(* Logix 5000 AddOnInstructionDefinition export Banner_LTF_Param_v4; software revision 33.00 *)

TYPE Banner_IOL_Port_v4 :   // UDT that has all of the data items necessary to communicate with a specific Port on a IO-Link Master
STRUCT
   Port_Controlled : INT;   // Each bit represents a port on an IO-Link Master. Set to 1 to tell AOI to control that port.
   Port_Activate : INT;   // Each bit represents a port on an IO-Link Master. When ON that port will process any commands in queue.
   Port_Read : INT;   // Each bit represents a port on an IO-Link Master. Used to determine when device AOI has requested a Read command.
   Port_Write : INT;   // Each bit represents a port on an IO-Link Master. Used to determine when device AOI has requested a Write command.
   Port_RW_Complete : INT;   // Each bit represents a port on an IO-Link Master. Tells device AOI that Read or Write request has been completed.
   Port_Device_Read : INT;
   Data_Transfer : SINT[190];   // Array to transfer data from IO-Master to device AOIs.
END_STRUCT
END_TYPE

TYPE Banner_LTF_RD_v4 :   // UDT with all of the Read only parameters for LTF.
STRUCT
   Master_Cycle_Time : INT;
   Min_Cycle_Time : INT;
   M_Sequence_Capability : INT;
   IO_Link_Version_ID : INT;
   Process_Data_Input_Length : INT;
   Process_Data_Output_Length : INT;
   Combined_Vendor_ID : DINT;   // IO-Link Vendor ID
   Vendor_ID1 : INT;
   Vendor_ID2 : INT;
   Combined_Device_ID : DINT;   // IO-Link Device ID
   Device_ID1 : INT;
   Device_ID2 : INT;
   Device_ID3 : INT;
   Serial_Number : STRING;
   Teach_State : SINT;   // 0 =IDLE, 1 = SP1 Success, 4 = Wait for Command, 5 = Busy, 7 = Error
   SP1_TP1 : SINT;   // 0 = not taught or unsuccessful, 1 = successfully taught
   SP2_TP2 : SINT;   // 0 = not taught or unsuccessful, 1 = successfully taught
   Measurement_Value : DINT;   // Measurement value in .1 mm.
   Excess_Gain_Percent : DINT;   // Excess gain expressed as a percentage of minimum signal
   Stability : INT;   // 0 = No target exists, 1 = Marginal or multiple peaks, 2 = Stable
   Display_String : STRING;   // String currently being displayed on the LED display of the sensor
END_STRUCT
END_TYPE

TYPE Banner_LTF_v4 :   // UDT with all of the parameters for LTF.
STRUCT
   Initial_Global_Read : BOOL;   // Determines if all of the IO-Link data has been read into the PLC yet
   Command : INT;   // Value placed in here will activate a read or write to a specifc IO-Link Index
   Read_Data : Banner_LTF_RD_v4;   // Read Only Data
   Write_Data : Banner_LTF_WD_v4;   // Write Data
   Archive : Banner_LTF_WD_v4;   // Archive write data
   Reset : BOOL;   // Resets AOI. This will force a complete parameter read of the sensor.
END_STRUCT
END_TYPE

TYPE Banner_LTF_WD_v4 :   // UDT that stores the Write Data for a LTF.
STRUCT
   System_Command : INT;   // See IODD file for list of commands that can be activated via the System Command interface
   Parameter_Access_Lock : SINT;   // Write access to all parameters is prohibited while value is 1. Only this parameter can be adjusted when value is 1.
   Data_Storage_Lock : SINT;   // Automatic data storage is disabled when this value is equal to 1. Read access is not affected.
   Local_Parameterization_Lock : SINT;   // Parameterization via local control elements on device is disabled.
   Local_User_Interface_Lock : SINT;   // Operation of local user interface is disabled.
   Teach_Channel : INT;   // 0 = Default, 1 = BDC1, 2 = BDC2
   BDC1_Setpoint_SP1 : DINT;   // SP1 switch point in Switch or Window mode. Range 500 to 120000 (.1 mm increments)
   BDC1_Setpoint_SP2 : DINT;   // SP2 switch point in Window mode only. Range 500 to 120000 (.1 mm increments)
   BDC1_Swithpoint_Logic : INT;   // Discrete output only. 0 = Light Operate, 1 = Dark Operate
   BDC1_BDC_Mode : INT;   // 1 = Switch Mode/Single Point Mode, 2 = Window Mode, 132 = Health(LO)/Alarm Mode(DO)
   BDC1_Hysteresis : DINT;   // 0 = Automatically set by sensor, 2-12000 = Manual (2 to 12000 mm)
   BDC2_Setpoint_SP1 : DINT;   // SP1 switch point in Switch or Window mode. Range 500 to 120000 (.1 mm increments)
   BDC2_Setpoint_SP2 : DINT;   // SP2 switch point in Window mode only. Range 500 to 120000 (.1 mm increments)
   BDC2_Switchpoint_Logic : INT;   // Discrete output only. 0 = Light Operate, 1 = Dark Operate
   BDC2_BDC_Mode : INT;   // 1 = Switch Mode/Single Point Mode, 2 = Window Mode, 132 = Health(LO)/Alarm Mode(DO), 133 Pulse Frequency Modulation
   BDC2_Hysteresis : DINT;   // 0 = Automatically set by sensor, 2-12000 = Manual (2 to 12000 mm)
   Response_Speed : INT;   // 0 = Fast, 1 = Standard, 2 = Medium, 3 = Slow
   Zero_Reference_Location : INT;   // 0 = Near, 1 = Far
   Shift_Zero_Reference_After_Teach : INT;   // 0 = Off, 1 = AutoSet, 2 = SetZero
   Sensor_Lockout : SINT;   // 0 = No Lock Out, 1 = Sensor Locked
   Output_Polarity : SINT;   // 0 = PNP, 1 = NPN
   IOL_Filter_Time : DINT;   // Time to average IOL process data measurement between updates. 0 to 65535 ms.
   Display_Read : SINT;   // 0 = Nomral, 1 = Inverted
   Display_Units : SINT;   // 0 = mm, 1 = inches
   Display_Sleep : SINT;   // 0 = 1 min, 1 = 5 min, 2 = 15 min, 3 = 60 min, 4 = Disabled
   Remote_Input_Type : SINT;   // 0 = Teach, 1 = Laser Enable, 2 = Sync Master, 3 = Sync Slave, 4 = Disabled
   BDC1_Delay_Mode : INT;   // 0 = Delay timer disabled, 1 = On & Off Delay, 2 = Off One-Shot timer, 3 = On One-Shot timer
   BDC1_Delay_On_OneShot_Delay : DINT;   // 0 to 9999 ms. 0 ms disables On delay or On/Off oneshot delay.
   BDC1_Delay_Off_OneShot_Delay : DINT;   // 0 to 9999 ms. 0 ms disables Off delay or On/Off oneshot delay.
   BDC1_Switch_Point_Reference : INT;   // 0 = Object, 1 = Background, 2 = Custom
   BDC1_User_Teach_Offset : DINT;   // The user selected teach offset. In Custom mode this value can be either + or -. In Object or Background mode this must be set to 0. Range -119500 to 119500 (-11950 to 11950 mm)
   BDC1_Midpoint_Window_Size : DINT;   // In Midpoint teach mode this will set the size of the window for midpoint teach. Default is 20 mm. Range 0 to 119500 (0 - 11950 mm).
   BDC1_Midpoint_Teach_Offset_Size : DINT;   // The offset value that is applied to a Midpoint teach. Range: -119500 to 119500 (-11950 to 11950 mm)
   BDC2_Delay_Mode : INT;   // 0 = Delay timer disabled, 1 = On & Off Delay, 2 = Off One-Shot timer, 3 = On One-Shot timer
   BDC2_Delay_On_OneShot_Delay : DINT;   // 0 to 9999. 0 ms disables On delay or On/Off oneshot delay.
   BDC2_Delay_Off_OneShot_Delay : DINT;   // 0 to 9999. 0 ms disables Off delay or On/Off oneshot delay.
   BDC2_Switch_Point_Reference : INT;   // 0 = Object, 1 = Background, 2 = Custom
   BDC2_User_Teach_Offset : DINT;   // The user selected teach offset. In Custom mode this value can be either + or -. In Object or Background mode this must be set to 0. Range: -119500 to 119500 (-11950 to 11950 mm).
   BDC2_Midpoint_Window_Size : DINT;   // In Midpoint teach mode this will set the size of the window for midpoint teach. Default is 20 mm. Range 0 to 119500 (0 - 11950 mm).
   BDC2_Midpoint_Teach_Offset_Size : DINT;   // The offset value that is applied to a Midpoint teach. Range: -119500 to 119500 (-11950 to 11950 mm).
   Near_Frequency : DINT;   // Frequency corresponding to a target at the near limit of the sensing range. Range 100 to 10000 Hz.
   Far_Frequency : DINT;   // Frequency corresponding to a target at the far limit of the sensing range. Range 100 to 10000 Hz.
END_STRUCT
END_TYPE

ADD_ON_INSTRUCTION Banner_LTF_Param_v4   (* revision 4.1, vendor Banner Engineering *)
// AOI to read and write parameter data to an IO-Link LTF.
VAR_IN_OUT
   LTF : Banner_LTF_v4; {required}
   Port_Data : Banner_IOL_Port_v4; {required}
END_VAR
VAR_INPUT
   Port : DINT; {required}
END_VAR
VAR
   Local_Control : DINT; {access None}
   Global_Read_Command_Value : INT; {access None}
   Global_Write_Command_Value : INT; {access None}
   Command_Being_Processed : BOOL; {access None}
   Update_Archive : BOOL; {access None}
   Index_Write_Control : DINT; {access None}
   Index_Write_Inprocess : INT; {access None}
   Inprocess_Index : DINT; {access None}
END_VAR

ROUTINE Logic   (* ladder *)
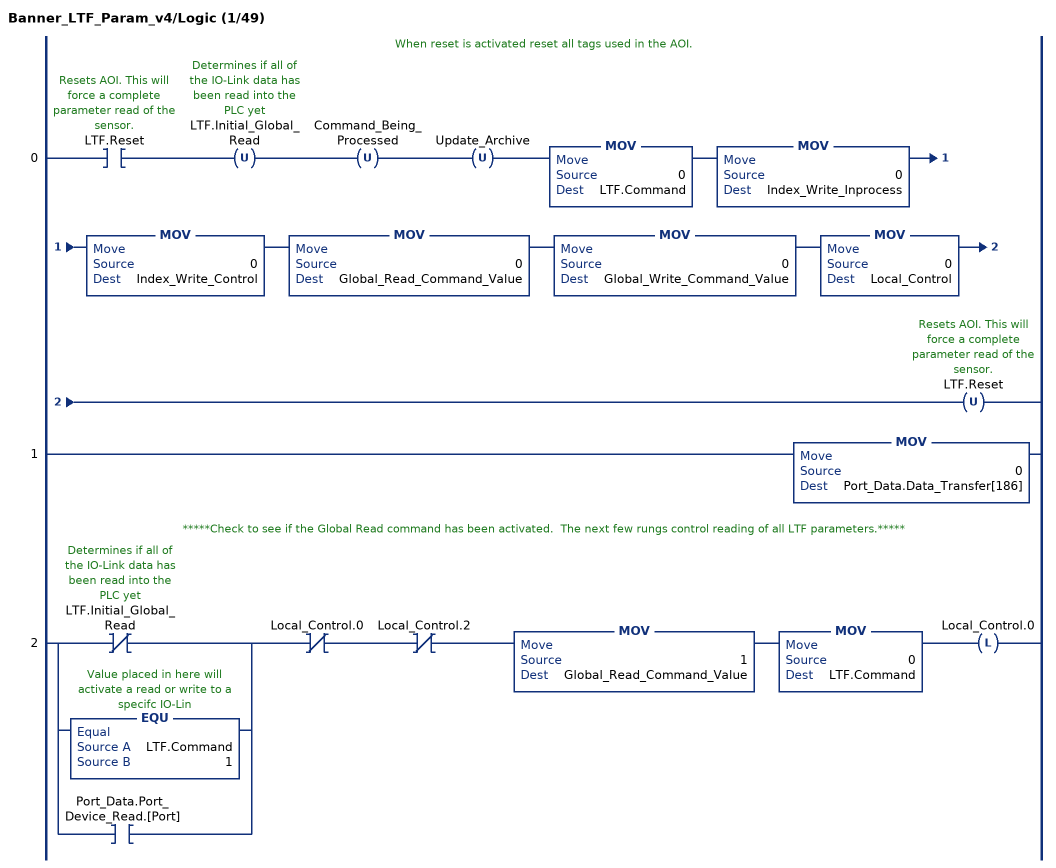
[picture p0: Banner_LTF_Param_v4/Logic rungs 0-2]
   // When reset is activated reset all tags used in the AOI.
   0: XIC(LTF.Reset)OTU(LTF.Initial_Global_Read)OTU(Command_Being_Processed)OTU(Update_Archive)MOV(0,LTF.Command)MOV(0,Index_Write_Inprocess)MOV(0,Index_Write_Control)MOV(0,Global_Read_Command_Value)MOV(0,Global_Write_Command_Value)MOV(0,Local_Control)OTU(LTF.Reset);
   1: MOV(0,Port_Data.Data_Transfer[186]);
   // *****Check to see if the Global Read command has been activated.  The next few rungs control reading of all LTF parameters.*****
   2: [XIO(LTF.Initial_Global_Read) ,EQU(LTF.Command,1) ,XIC(Port_Data.Port_Device_Read.[Port]) ]XIO(Local_Control.0)XIO(Local_Control.2)MOV(1,Global_Read_Command_Value)MOV(0,LTF.Command)OTL(Local_Control.0);
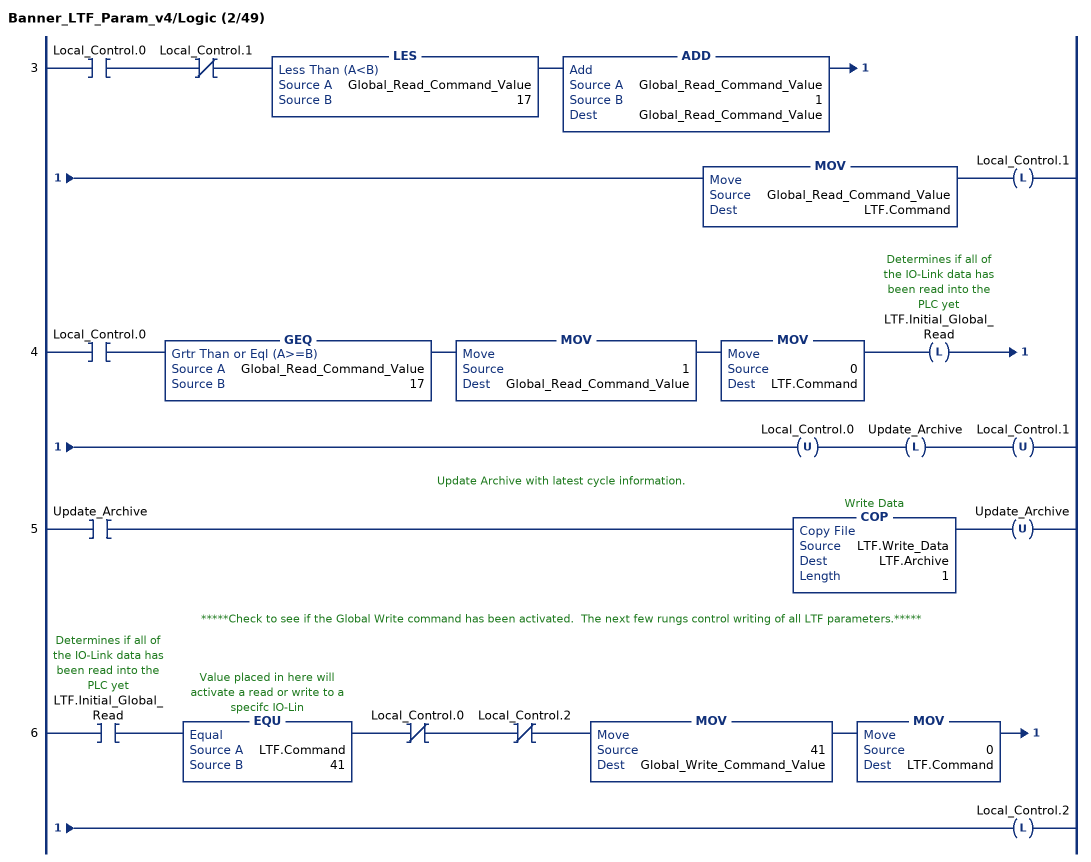
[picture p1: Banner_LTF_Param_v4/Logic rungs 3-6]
   3: XIC(Local_Control.0)XIO(Local_Control.1)LES(Global_Read_Command_Value,17)ADD(Global_Read_Command_Value,1,Global_Read_Command_Value)MOV(Global_Read_Command_Value,LTF.Command)OTL(Local_Control.1);
   4: XIC(Local_Control.0)GEQ(Global_Read_Command_Value,17)MOV(1,Global_Read_Command_Value)MOV(0,LTF.Command)OTL(LTF.Initial_Global_Read)OTU(Local_Control.0)OTL(Update_Archive)OTU(Local_Control.1);
   // Update Archive with latest cycle information.
   5: XIC(Update_Archive)COP(LTF.Write_Data,LTF.Archive,1)OTU(Update_Archive);
   // *****Check to see if the Global Write command has been activated.  The next few rungs control writing of all LTF parameters.*****
   6: XIC(LTF.Initial_Global_Read)EQU(LTF.Command,41)XIO(Local_Control.0)XIO(Local_Control.2)MOV(41,Global_Write_Command_Value)MOV(0,LTF.Command)OTL(Local_Control.2);
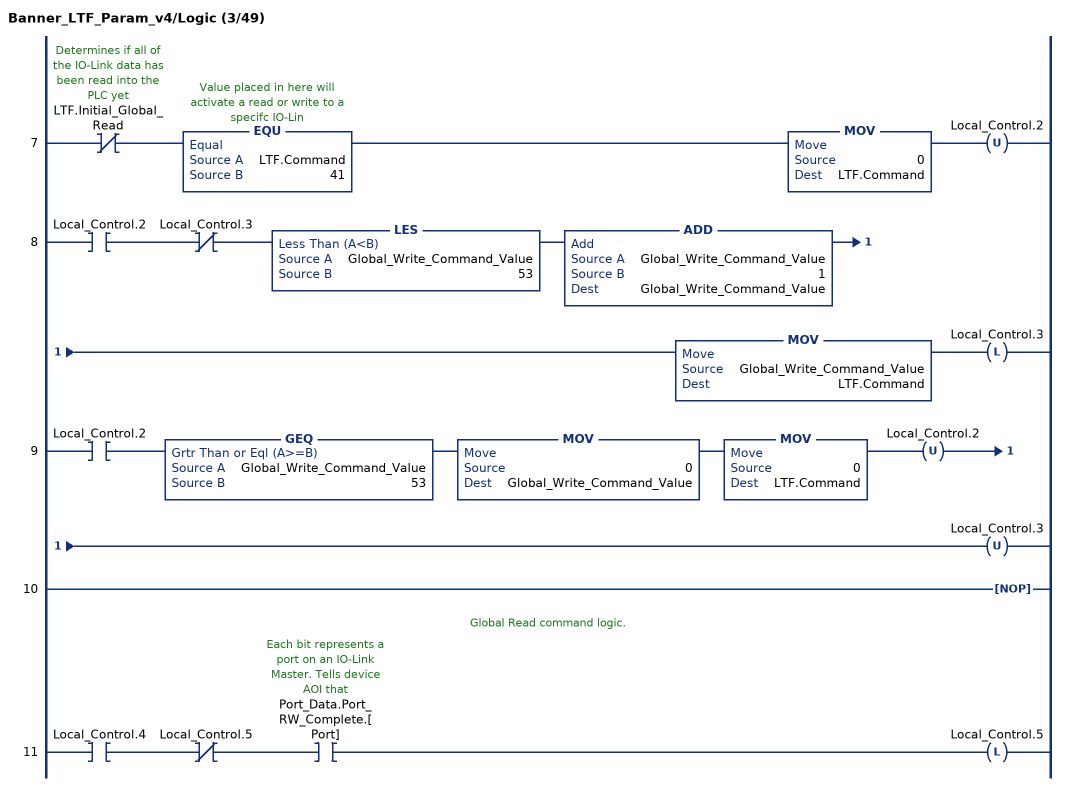
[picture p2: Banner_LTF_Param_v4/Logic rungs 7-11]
   7: XIO(LTF.Initial_Global_Read)EQU(LTF.Command,41)MOV(0,LTF.Command)OTU(Local_Control.2);
   8: XIC(Local_Control.2)XIO(Local_Control.3)LES(Global_Write_Command_Value,53)ADD(Global_Write_Command_Value,1,Global_Write_Command_Value)MOV(Global_Write_Command_Value,LTF.Command)OTL(Local_Control.3);
   9: XIC(Local_Control.2)GEQ(Global_Write_Command_Value,53)MOV(0,Global_Write_Command_Value)MOV(0,LTF.Command)OTU(Local_Control.2)OTU(Local_Control.3);
   10: NOP();
   // Global Read command logic.
   11: XIC(Local_Control.4)XIO(Local_Control.5)XIC(Port_Data.Port_RW_Complete.[Port])OTL(Local_Control.5);
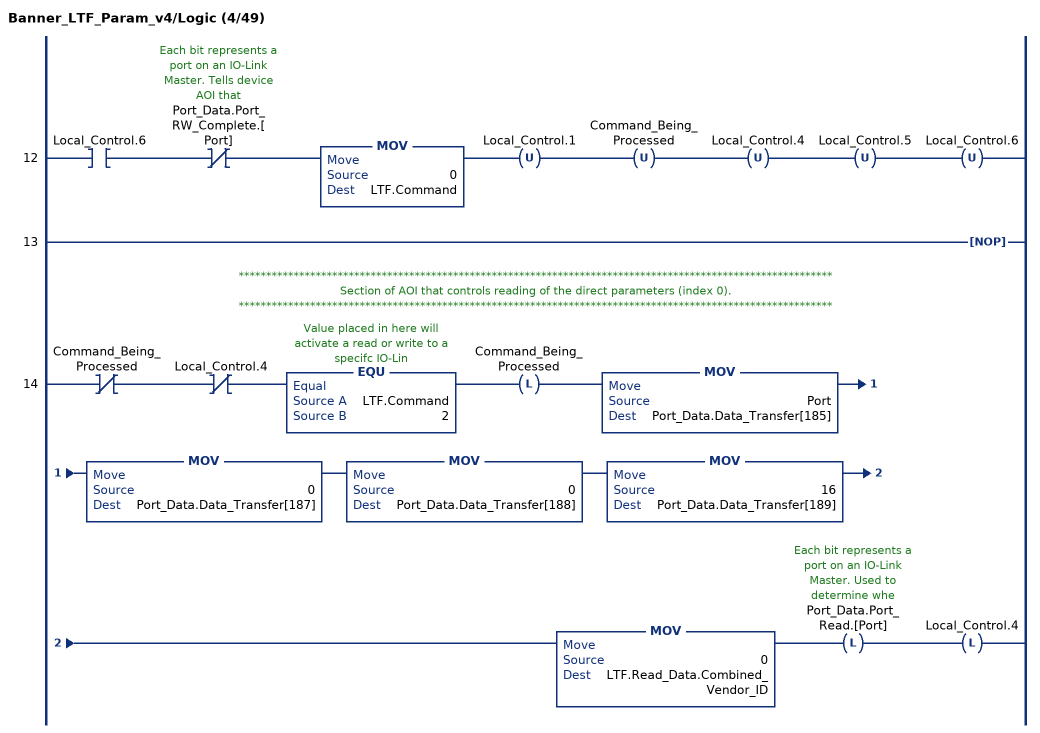
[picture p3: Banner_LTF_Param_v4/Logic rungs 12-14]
   12: XIC(Local_Control.6)XIO(Port_Data.Port_RW_Complete.[Port])MOV(0,LTF.Command)OTU(Local_Control.1)OTU(Command_Being_Processed)OTU(Local_Control.4)OTU(Local_Control.5)OTU(Local_Control.6);
   13: NOP();
   // ************************************************************************************************************
   // Section of AOI that controls reading of the direct parameters (index 0).
   // ************************************************************************************************************
   14: XIO(Command_Being_Processed)XIO(Local_Control.4)EQU(LTF.Command,2)OTL(Command_Being_Processed)MOV(Port,Port_Data.Data_Transfer[185])MOV(0,Port_Data.Data_Transfer[187])MOV(0,Port_Data.Data_Transfer[188])MOV(16,Port_Data.Data_Transfer[189])MOV(0,LTF.Read_Data.Combined_Vendor_ID)OTL(Port_Data.Port_Read.[Port])OTL(Local_Control.4);
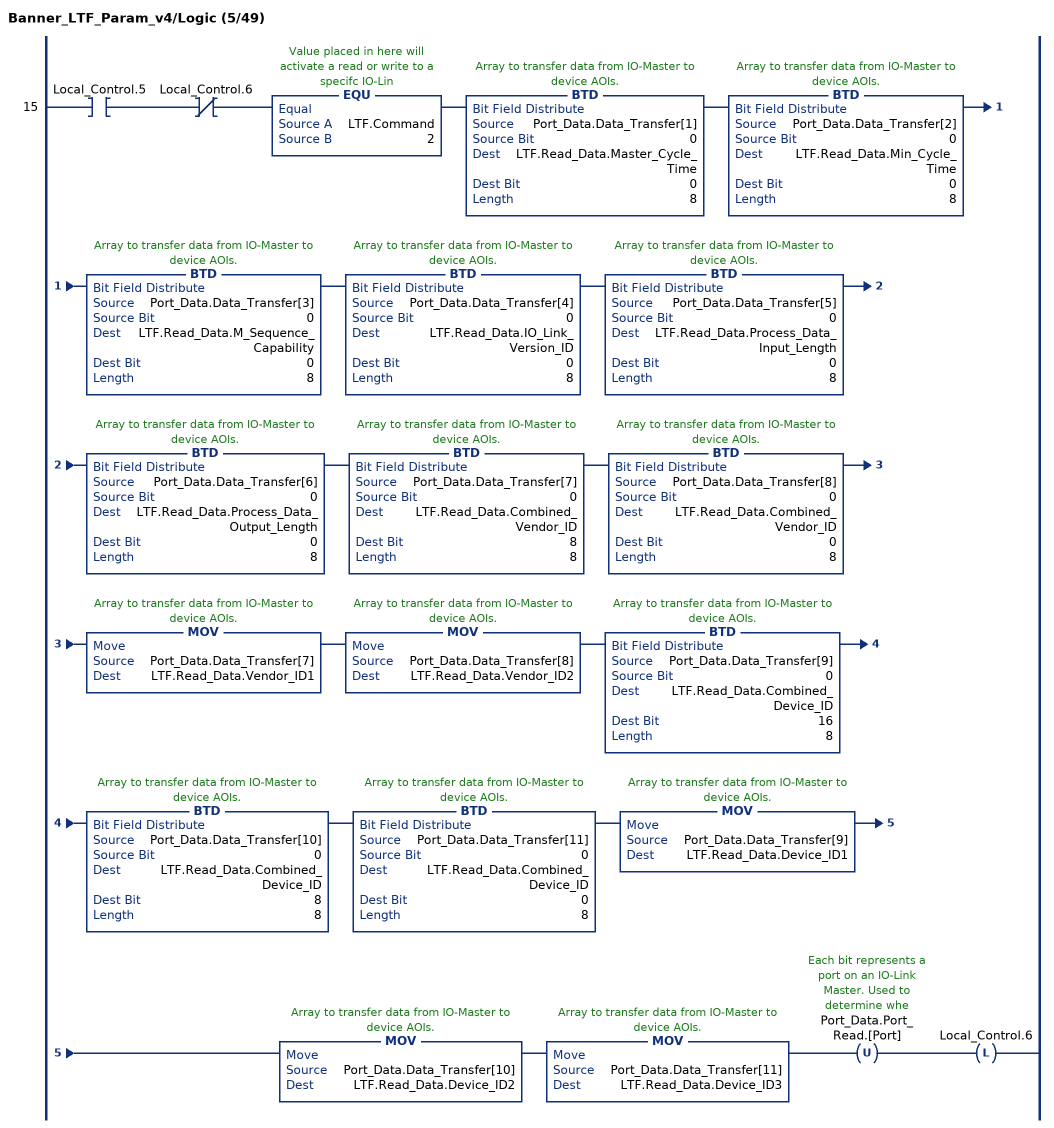
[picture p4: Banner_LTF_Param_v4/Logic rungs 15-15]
   15: XIC(Local_Control.5)XIO(Local_Control.6)EQU(LTF.Command,2)BTD(Port_Data.Data_Transfer[1],0,LTF.Read_Data.Master_Cycle_Time,0,8)BTD(Port_Data.Data_Transfer[2],0,LTF.Read_Data.Min_Cycle_Time,0,8)BTD(Port_Data.Data_Transfer[3],0,LTF.Read_Data.M_Sequence_Capability,0,8)BTD(Port_Data.Data_Transfer[4],0,LTF.Read_Data.IO_Link_Version_ID,0,8)BTD(Port_Data.Data_Transfer[5],0,LTF.Read_Data.Process_Data_Input_Length,0,8)BTD(Port_Data.Data_Transfer[6],0,LTF.Read_Data.Process_Data_Output_Length,0,8)BTD(Port_Data.Data_Transfer[7],0,LTF.Read_Data.Combined_Vendor_ID,8,8)BTD(Port_Data.Data_Transfer[8],0,LTF.Read_Data.Combined_Vendor_ID,0,8)MOV(Port_Data.Data_Transfer[7],LTF.Read_Data.Vendor_ID1)MOV(Port_Data.Data_Transfer[8],LTF.Read_Data.Vendor_ID2)BTD(Port_Data.Data_Transfer[9],0,LTF.Read_Data.Combined_Device_ID,16,8)BTD(Port_Data.Data_Transfer[10],0,LTF.Read_Data.Combined_Device_ID,8,8)BTD(Port_Data.Data_Transfer[11],0,LTF.Read_Data.Combined_Device_ID,0,8)MOV(Port_Data.Data_Transfer[9],LTF.Read_Data.Device_ID1)MOV(Port_Data.Data_Transfer[10],LTF.Read_Data.Device_ID2)MOV(Port_Data.Data_Transfer[11],LTF.Read_Data.Device_ID3)OTU(Port_Data.Port_Read.[Port])OTL(Local_Control.6);
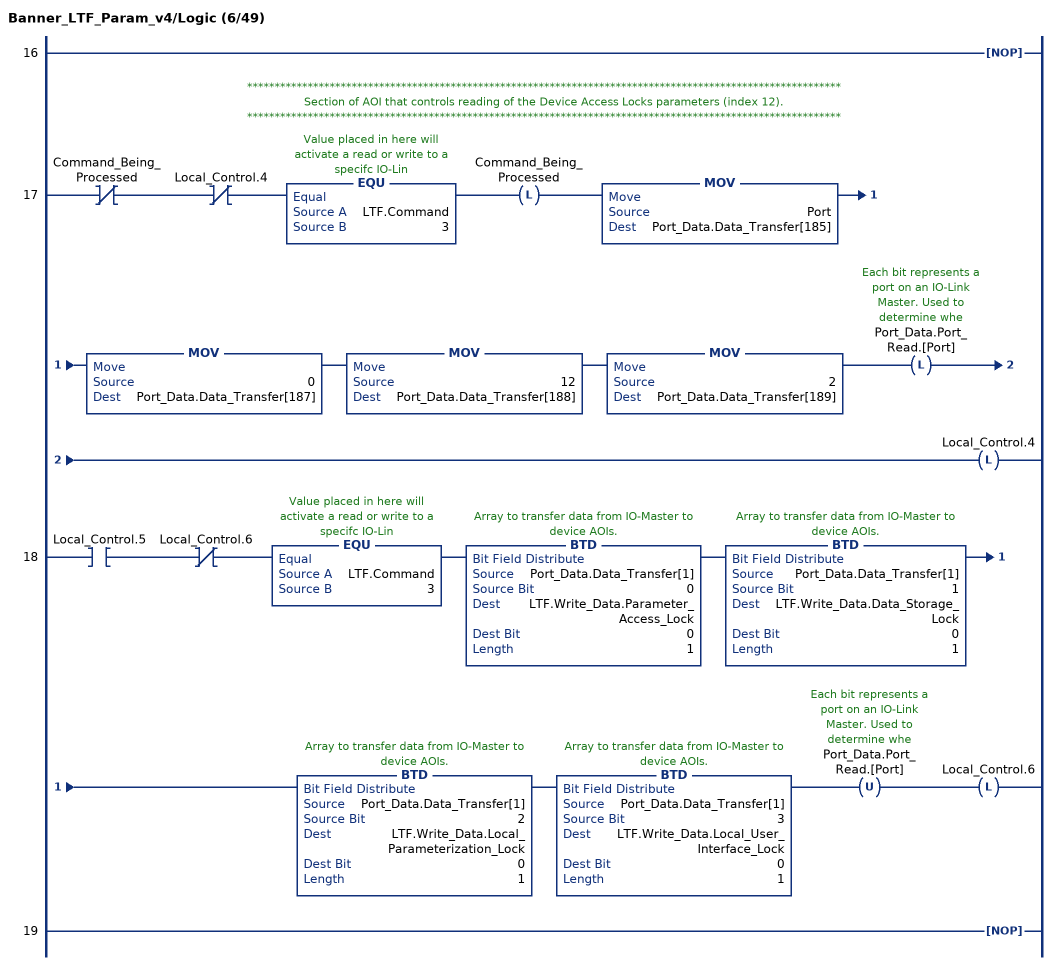
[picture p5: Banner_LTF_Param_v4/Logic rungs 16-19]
   16: NOP();
   // ************************************************************************************************************
   // Section of AOI that controls reading of the Device Access Locks parameters (index 12).
   // ************************************************************************************************************
   17: XIO(Command_Being_Processed)XIO(Local_Control.4)EQU(LTF.Command,3)OTL(Command_Being_Processed)MOV(Port,Port_Data.Data_Transfer[185])MOV(0,Port_Data.Data_Transfer[187])MOV(12,Port_Data.Data_Transfer[188])MOV(2,Port_Data.Data_Transfer[189])OTL(Port_Data.Port_Read.[Port])OTL(Local_Control.4);
   18: XIC(Local_Control.5)XIO(Local_Control.6)EQU(LTF.Command,3)BTD(Port_Data.Data_Transfer[1],0,LTF.Write_Data.Parameter_Access_Lock,0,1)BTD(Port_Data.Data_Transfer[1],1,LTF.Write_Data.Data_Storage_Lock,0,1)BTD(Port_Data.Data_Transfer[1],2,LTF.Write_Data.Local_Parameterization_Lock,0,1)BTD(Port_Data.Data_Transfer[1],3,LTF.Write_Data.Local_User_Interface_Lock,0,1)OTU(Port_Data.Port_Read.[Port])OTL(Local_Control.6);
   19: NOP();
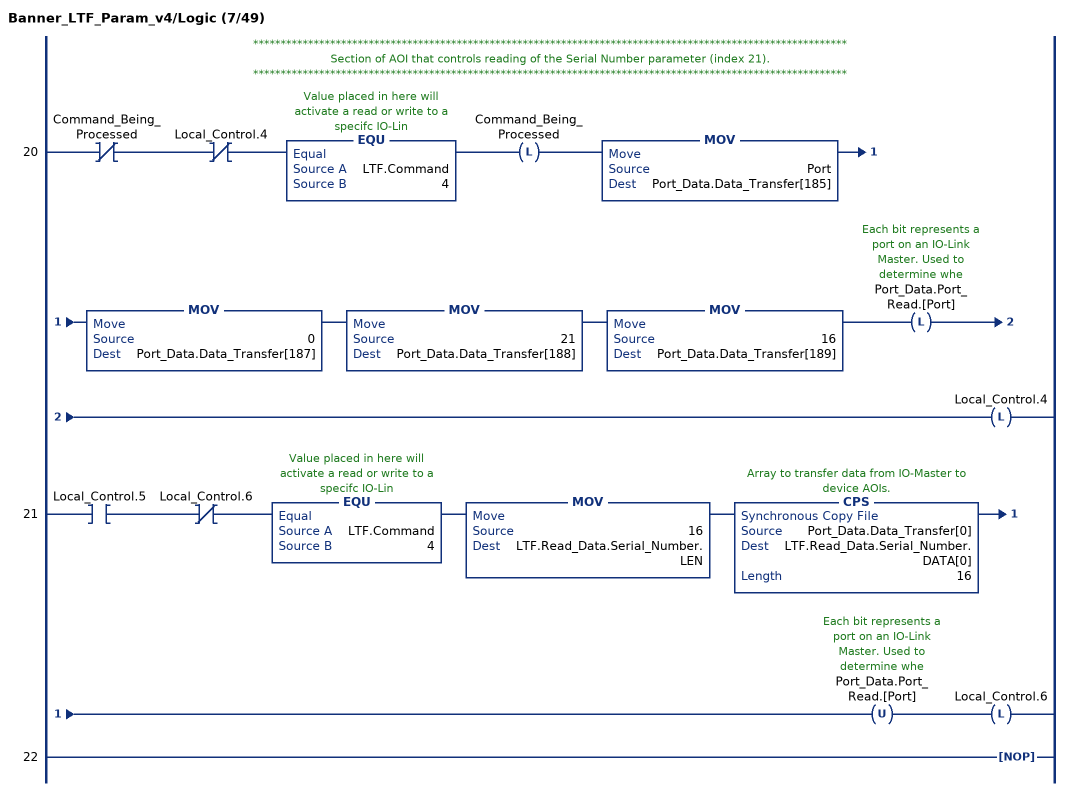
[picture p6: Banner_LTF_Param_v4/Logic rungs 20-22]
   // ************************************************************************************************************
   // Section of AOI that controls reading of the Serial Number parameter (index 21).
   // ************************************************************************************************************
   20: XIO(Command_Being_Processed)XIO(Local_Control.4)EQU(LTF.Command,4)OTL(Command_Being_Processed)MOV(Port,Port_Data.Data_Transfer[185])MOV(0,Port_Data.Data_Transfer[187])MOV(21,Port_Data.Data_Transfer[188])MOV(16,Port_Data.Data_Transfer[189])OTL(Port_Data.Port_Read.[Port])OTL(Local_Control.4);
   21: XIC(Local_Control.5)XIO(Local_Control.6)EQU(LTF.Command,4)MOV(16,LTF.Read_Data.Serial_Number.LEN)CPS(Port_Data.Data_Transfer[0],LTF.Read_Data.Serial_Number.DATA[0],16)OTU(Port_Data.Port_Read.[Port])OTL(Local_Control.6);
   22: NOP();
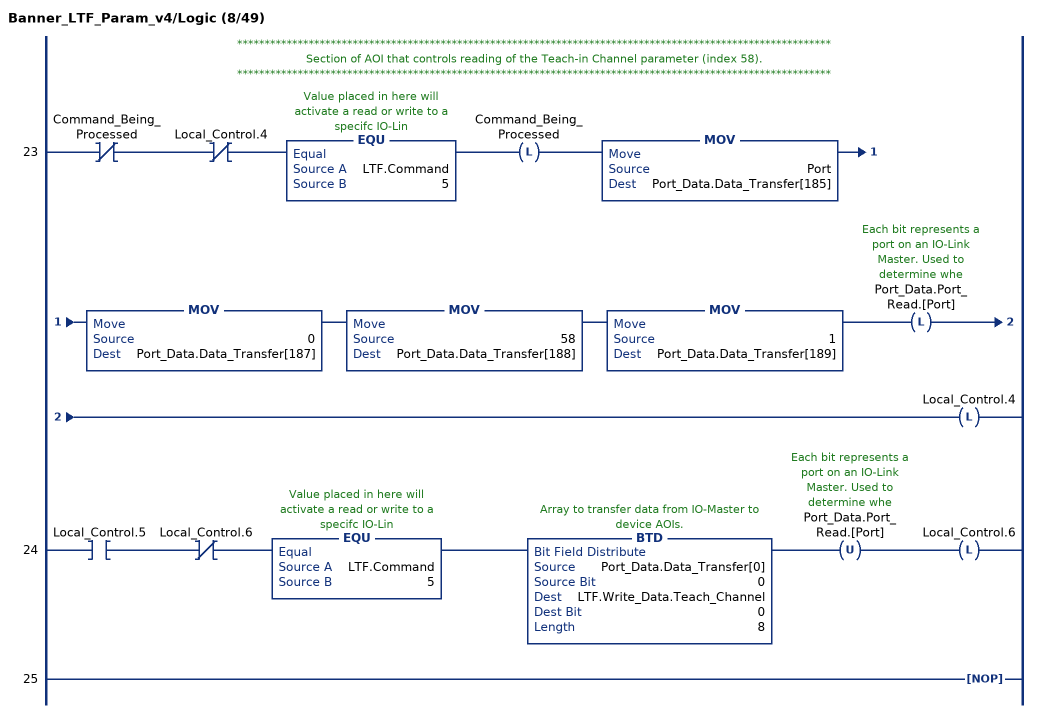
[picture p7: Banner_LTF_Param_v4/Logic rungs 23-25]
   // ************************************************************************************************************
   // Section of AOI that controls reading of the Teach-in Channel parameter (index 58).
   // ************************************************************************************************************
   23: XIO(Command_Being_Processed)XIO(Local_Control.4)EQU(LTF.Command,5)OTL(Command_Being_Processed)MOV(Port,Port_Data.Data_Transfer[185])MOV(0,Port_Data.Data_Transfer[187])MOV(58,Port_Data.Data_Transfer[188])MOV(1,Port_Data.Data_Transfer[189])OTL(Port_Data.Port_Read.[Port])OTL(Local_Control.4);
   24: XIC(Local_Control.5)XIO(Local_Control.6)EQU(LTF.Command,5)BTD(Port_Data.Data_Transfer[0],0,LTF.Write_Data.Teach_Channel,0,8)OTU(Port_Data.Port_Read.[Port])OTL(Local_Control.6);
   25: NOP();
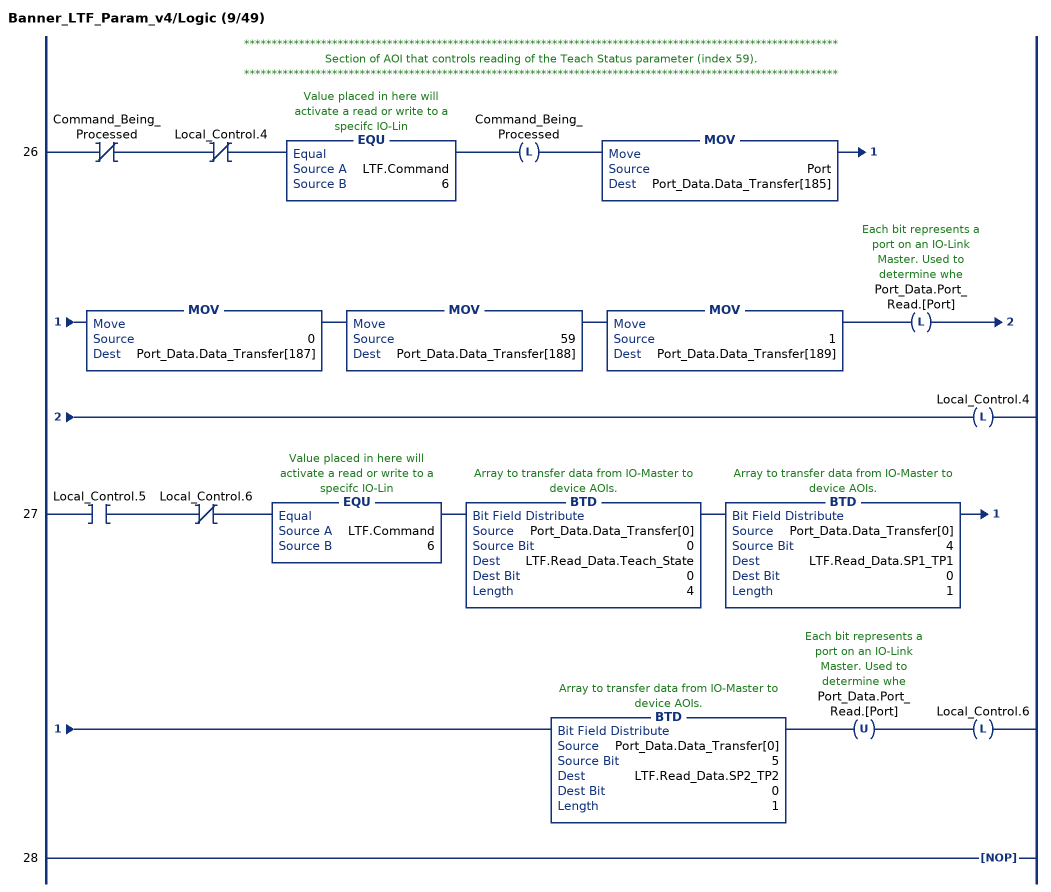
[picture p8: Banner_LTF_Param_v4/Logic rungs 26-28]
   // ************************************************************************************************************
   // Section of AOI that controls reading of the Teach Status parameter (index 59).
   // ************************************************************************************************************
   26: XIO(Command_Being_Processed)XIO(Local_Control.4)EQU(LTF.Command,6)OTL(Command_Being_Processed)MOV(Port,Port_Data.Data_Transfer[185])MOV(0,Port_Data.Data_Transfer[187])MOV(59,Port_Data.Data_Transfer[188])MOV(1,Port_Data.Data_Transfer[189])OTL(Port_Data.Port_Read.[Port])OTL(Local_Control.4);
   27: XIC(Local_Control.5)XIO(Local_Control.6)EQU(LTF.Command,6)BTD(Port_Data.Data_Transfer[0],0,LTF.Read_Data.Teach_State,0,4)BTD(Port_Data.Data_Transfer[0],4,LTF.Read_Data.SP1_TP1,0,1)BTD(Port_Data.Data_Transfer[0],5,LTF.Read_Data.SP2_TP2,0,1)OTU(Port_Data.Port_Read.[Port])OTL(Local_Control.6);
   28: NOP();
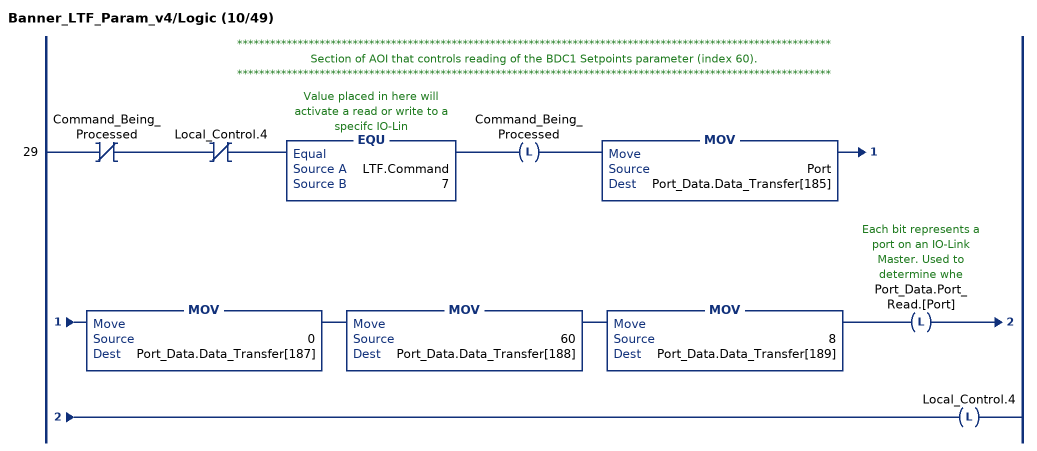
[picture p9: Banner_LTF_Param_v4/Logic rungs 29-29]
   // ************************************************************************************************************
   // Section of AOI that controls reading of the BDC1 Setpoints parameter (index 60).
   // ************************************************************************************************************
   29: XIO(Command_Being_Processed)XIO(Local_Control.4)EQU(LTF.Command,7)OTL(Command_Being_Processed)MOV(Port,Port_Data.Data_Transfer[185])MOV(0,Port_Data.Data_Transfer[187])MOV(60,Port_Data.Data_Transfer[188])MOV(8,Port_Data.Data_Transfer[189])OTL(Port_Data.Port_Read.[Port])OTL(Local_Control.4);
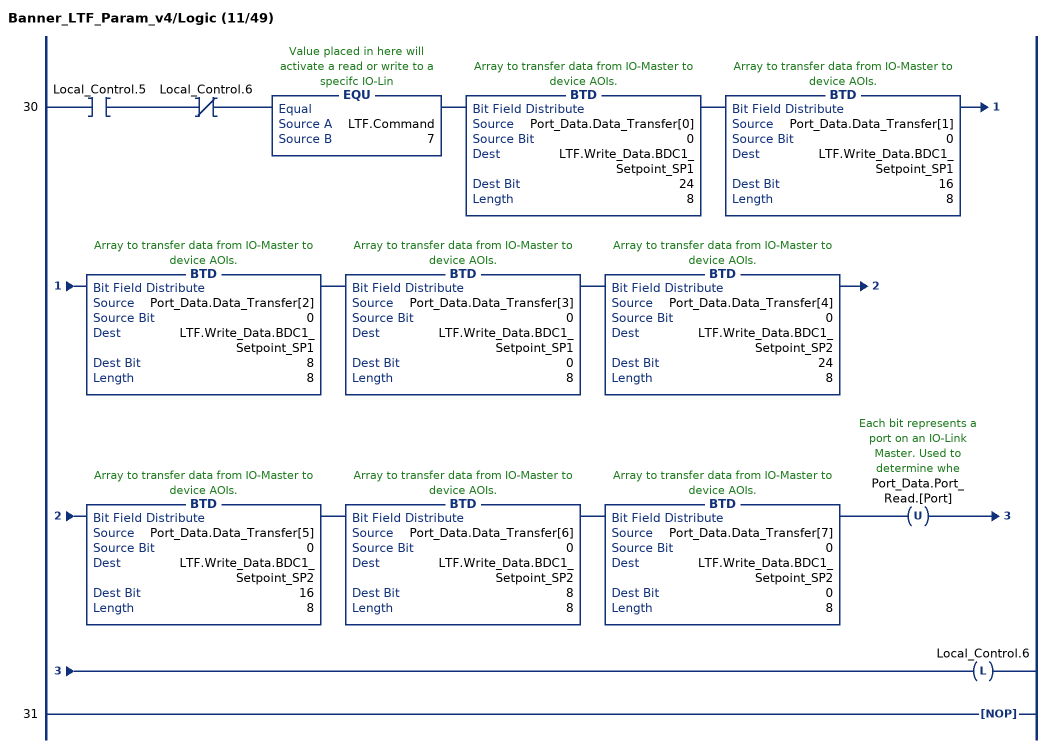
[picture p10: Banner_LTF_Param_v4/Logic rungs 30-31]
   30: XIC(Local_Control.5)XIO(Local_Control.6)EQU(LTF.Command,7)BTD(Port_Data.Data_Transfer[0],0,LTF.Write_Data.BDC1_Setpoint_SP1,24,8)BTD(Port_Data.Data_Transfer[1],0,LTF.Write_Data.BDC1_Setpoint_SP1,16,8)BTD(Port_Data.Data_Transfer[2],0,LTF.Write_Data.BDC1_Setpoint_SP1,8,8)BTD(Port_Data.Data_Transfer[3],0,LTF.Write_Data.BDC1_Setpoint_SP1,0,8)BTD(Port_Data.Data_Transfer[4],0,LTF.Write_Data.BDC1_Setpoint_SP2,24,8)BTD(Port_Data.Data_Transfer[5],0,LTF.Write_Data.BDC1_Setpoint_SP2,16,8)BTD(Port_Data.Data_Transfer[6],0,LTF.Write_Data.BDC1_Setpoint_SP2,8,8)BTD(Port_Data.Data_Transfer[7],0,LTF.Write_Data.BDC1_Setpoint_SP2,0,8)OTU(Port_Data.Port_Read.[Port])OTL(Local_Control.6);
   31: NOP();
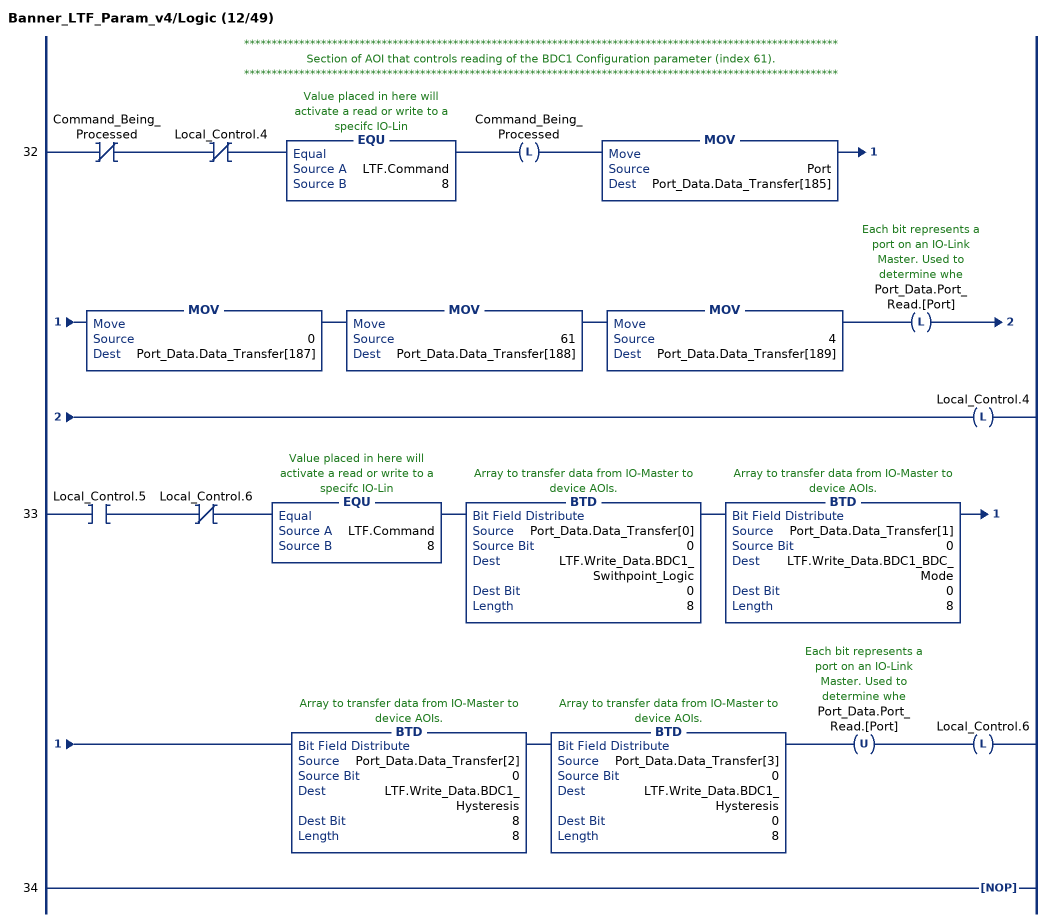
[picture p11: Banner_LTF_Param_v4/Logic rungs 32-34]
   // ************************************************************************************************************
   // Section of AOI that controls reading of the BDC1 Configuration parameter (index 61).
   // ************************************************************************************************************
   32: XIO(Command_Being_Processed)XIO(Local_Control.4)EQU(LTF.Command,8)OTL(Command_Being_Processed)MOV(Port,Port_Data.Data_Transfer[185])MOV(0,Port_Data.Data_Transfer[187])MOV(61,Port_Data.Data_Transfer[188])MOV(4,Port_Data.Data_Transfer[189])OTL(Port_Data.Port_Read.[Port])OTL(Local_Control.4);
   33: XIC(Local_Control.5)XIO(Local_Control.6)EQU(LTF.Command,8)BTD(Port_Data.Data_Transfer[0],0,LTF.Write_Data.BDC1_Swithpoint_Logic,0,8)BTD(Port_Data.Data_Transfer[1],0,LTF.Write_Data.BDC1_BDC_Mode,0,8)BTD(Port_Data.Data_Transfer[2],0,LTF.Write_Data.BDC1_Hysteresis,8,8)BTD(Port_Data.Data_Transfer[3],0,LTF.Write_Data.BDC1_Hysteresis,0,8)OTU(Port_Data.Port_Read.[Port])OTL(Local_Control.6);
   34: NOP();
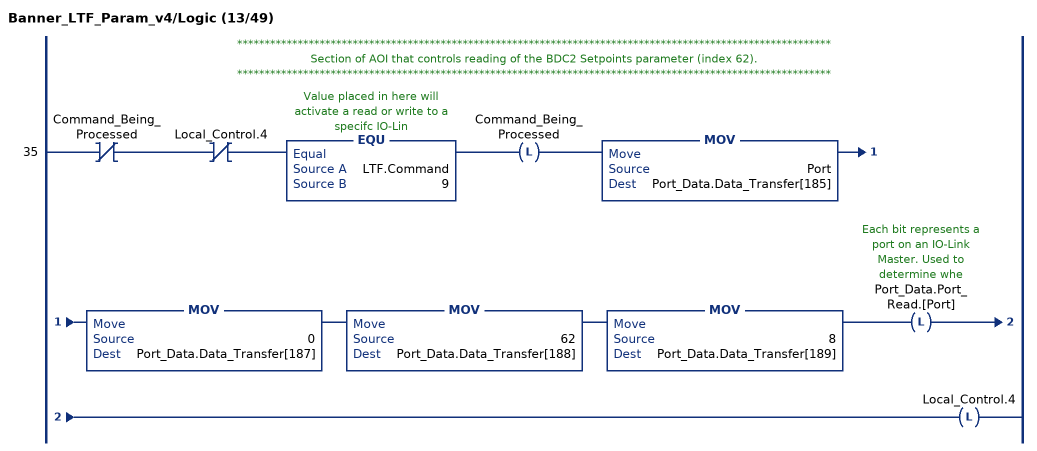
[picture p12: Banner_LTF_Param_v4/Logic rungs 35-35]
   // ************************************************************************************************************
   // Section of AOI that controls reading of the BDC2 Setpoints parameter (index 62).
   // ************************************************************************************************************
   35: XIO(Command_Being_Processed)XIO(Local_Control.4)EQU(LTF.Command,9)OTL(Command_Being_Processed)MOV(Port,Port_Data.Data_Transfer[185])MOV(0,Port_Data.Data_Transfer[187])MOV(62,Port_Data.Data_Transfer[188])MOV(8,Port_Data.Data_Transfer[189])OTL(Port_Data.Port_Read.[Port])OTL(Local_Control.4);
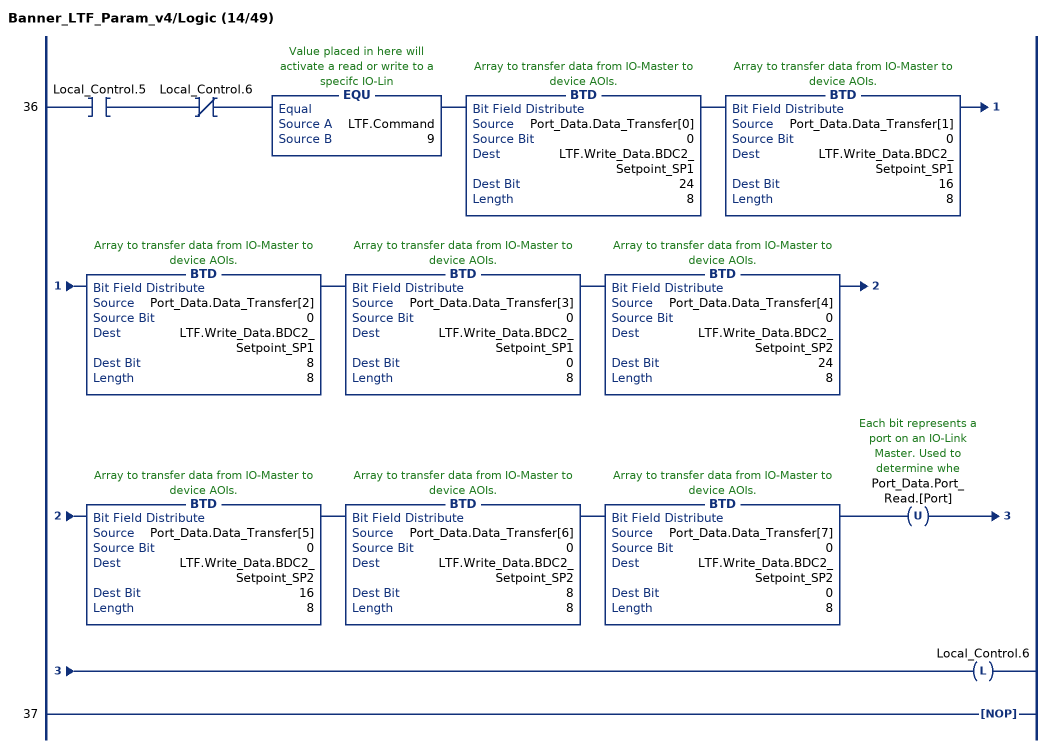
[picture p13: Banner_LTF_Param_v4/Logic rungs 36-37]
   36: XIC(Local_Control.5)XIO(Local_Control.6)EQU(LTF.Command,9)BTD(Port_Data.Data_Transfer[0],0,LTF.Write_Data.BDC2_Setpoint_SP1,24,8)BTD(Port_Data.Data_Transfer[1],0,LTF.Write_Data.BDC2_Setpoint_SP1,16,8)BTD(Port_Data.Data_Transfer[2],0,LTF.Write_Data.BDC2_Setpoint_SP1,8,8)BTD(Port_Data.Data_Transfer[3],0,LTF.Write_Data.BDC2_Setpoint_SP1,0,8)BTD(Port_Data.Data_Transfer[4],0,LTF.Write_Data.BDC2_Setpoint_SP2,24,8)BTD(Port_Data.Data_Transfer[5],0,LTF.Write_Data.BDC2_Setpoint_SP2,16,8)BTD(Port_Data.Data_Transfer[6],0,LTF.Write_Data.BDC2_Setpoint_SP2,8,8)BTD(Port_Data.Data_Transfer[7],0,LTF.Write_Data.BDC2_Setpoint_SP2,0,8)OTU(Port_Data.Port_Read.[Port])OTL(Local_Control.6);
   37: NOP();
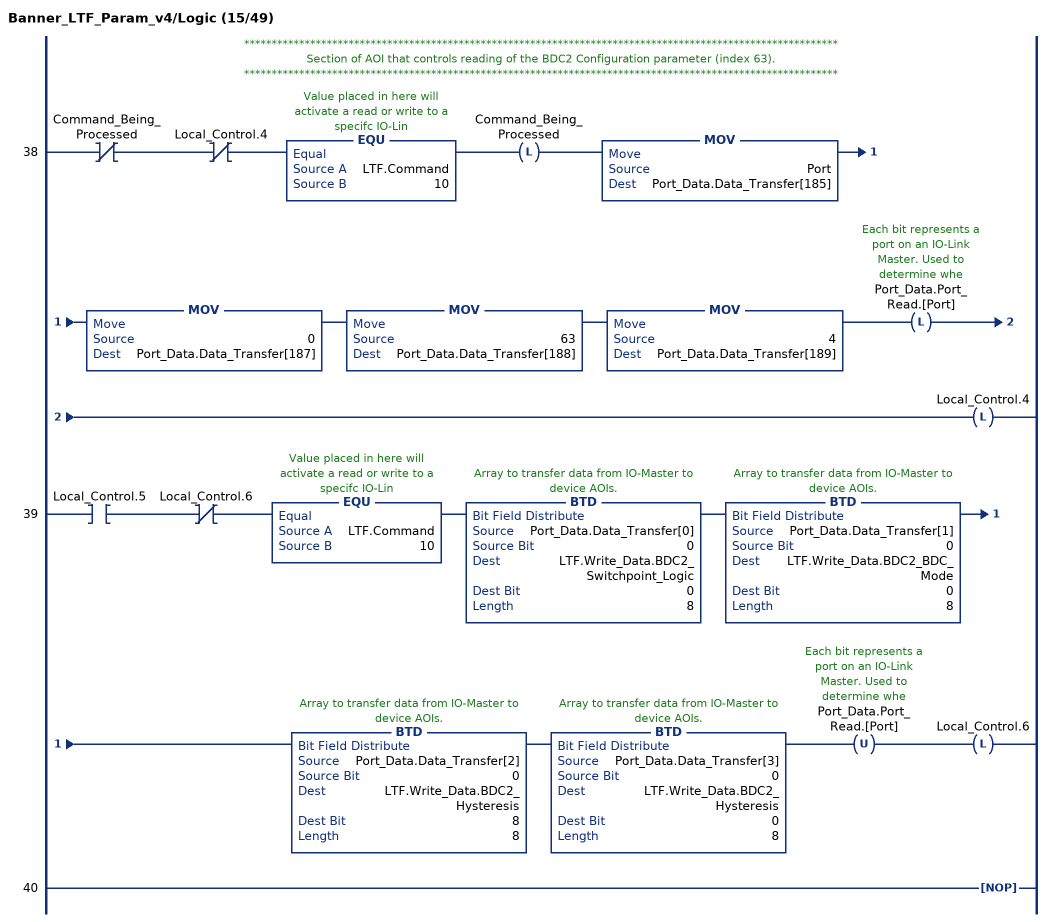
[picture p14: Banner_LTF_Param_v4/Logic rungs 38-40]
   // ************************************************************************************************************
   // Section of AOI that controls reading of the BDC2 Configuration parameter (index 63).
   // ************************************************************************************************************
   38: XIO(Command_Being_Processed)XIO(Local_Control.4)EQU(LTF.Command,10)OTL(Command_Being_Processed)MOV(Port,Port_Data.Data_Transfer[185])MOV(0,Port_Data.Data_Transfer[187])MOV(63,Port_Data.Data_Transfer[188])MOV(4,Port_Data.Data_Transfer[189])OTL(Port_Data.Port_Read.[Port])OTL(Local_Control.4);
   39: XIC(Local_Control.5)XIO(Local_Control.6)EQU(LTF.Command,10)BTD(Port_Data.Data_Transfer[0],0,LTF.Write_Data.BDC2_Switchpoint_Logic,0,8)BTD(Port_Data.Data_Transfer[1],0,LTF.Write_Data.BDC2_BDC_Mode,0,8)BTD(Port_Data.Data_Transfer[2],0,LTF.Write_Data.BDC2_Hysteresis,8,8)BTD(Port_Data.Data_Transfer[3],0,LTF.Write_Data.BDC2_Hysteresis,0,8)OTU(Port_Data.Port_Read.[Port])OTL(Local_Control.6);
   40: NOP();
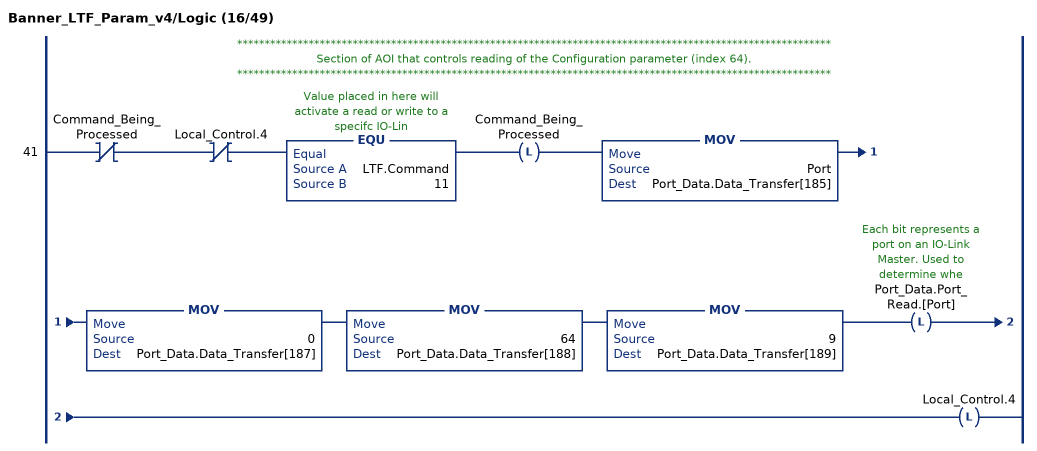
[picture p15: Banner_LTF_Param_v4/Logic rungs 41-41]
   // ************************************************************************************************************
   // Section of AOI that controls reading of the Configuration parameter (index 64).
   // ************************************************************************************************************
   41: XIO(Command_Being_Processed)XIO(Local_Control.4)EQU(LTF.Command,11)OTL(Command_Being_Processed)MOV(Port,Port_Data.Data_Transfer[185])MOV(0,Port_Data.Data_Transfer[187])MOV(64,Port_Data.Data_Transfer[188])MOV(9,Port_Data.Data_Transfer[189])OTL(Port_Data.Port_Read.[Port])OTL(Local_Control.4);
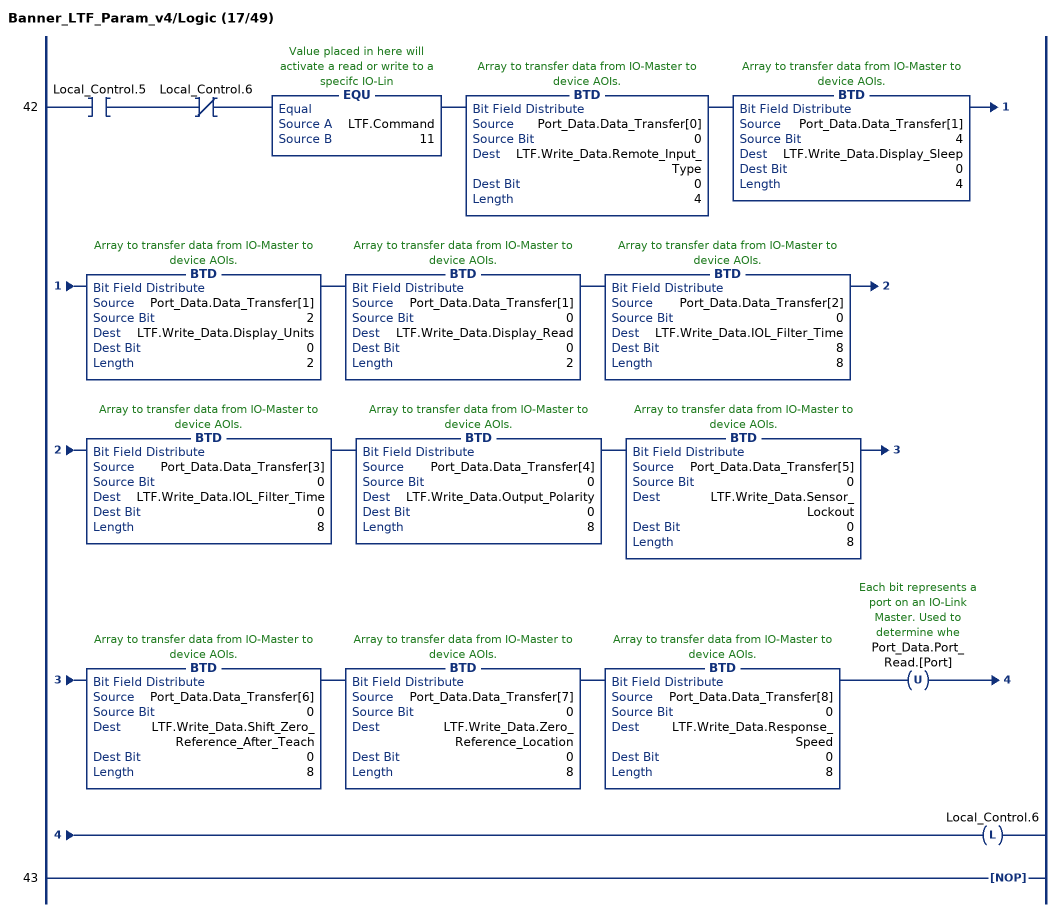
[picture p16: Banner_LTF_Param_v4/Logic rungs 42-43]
   42: XIC(Local_Control.5)XIO(Local_Control.6)EQU(LTF.Command,11)BTD(Port_Data.Data_Transfer[0],0,LTF.Write_Data.Remote_Input_Type,0,4)BTD(Port_Data.Data_Transfer[1],4,LTF.Write_Data.Display_Sleep,0,4)BTD(Port_Data.Data_Transfer[1],2,LTF.Write_Data.Display_Units,0,2)BTD(Port_Data.Data_Transfer[1],0,LTF.Write_Data.Display_Read,0,2)BTD(Port_Data.Data_Transfer[2],0,LTF.Write_Data.IOL_Filter_Time,8,8)BTD(Port_Data.Data_Transfer[3],0,LTF.Write_Data.IOL_Filter_Time,0,8)BTD(Port_Data.Data_Transfer[4],0,LTF.Write_Data.Output_Polarity,0,8)BTD(Port_Data.Data_Transfer[5],0,LTF.Write_Data.Sensor_Lockout,0,8)BTD(Port_Data.Data_Transfer[6],0,LTF.Write_Data.Shift_Zero_Reference_After_Teach,0,8)BTD(Port_Data.Data_Transfer[7],0,LTF.Write_Data.Zero_Reference_Location,0,8)BTD(Port_Data.Data_Transfer[8],0,LTF.Write_Data.Response_Speed,0,8)OTU(Port_Data.Port_Read.[Port])OTL(Local_Control.6);
   43: NOP();
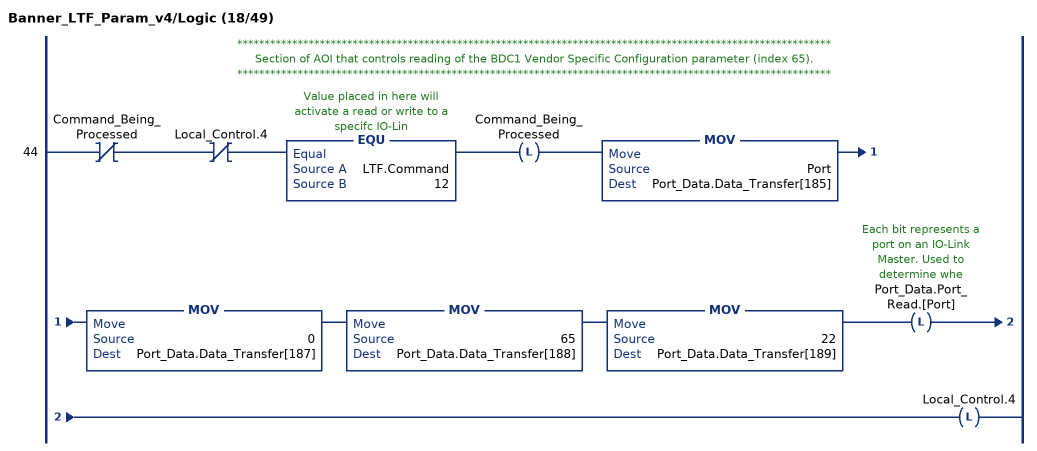
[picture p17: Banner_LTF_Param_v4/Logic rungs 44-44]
   // ************************************************************************************************************
   // Section of AOI that controls reading of the BDC1 Vendor Specific Configuration parameter (index 65).
   // ************************************************************************************************************
   44: XIO(Command_Being_Processed)XIO(Local_Control.4)EQU(LTF.Command,12)OTL(Command_Being_Processed)MOV(Port,Port_Data.Data_Transfer[185])MOV(0,Port_Data.Data_Transfer[187])MOV(65,Port_Data.Data_Transfer[188])MOV(22,Port_Data.Data_Transfer[189])OTL(Port_Data.Port_Read.[Port])OTL(Local_Control.4);
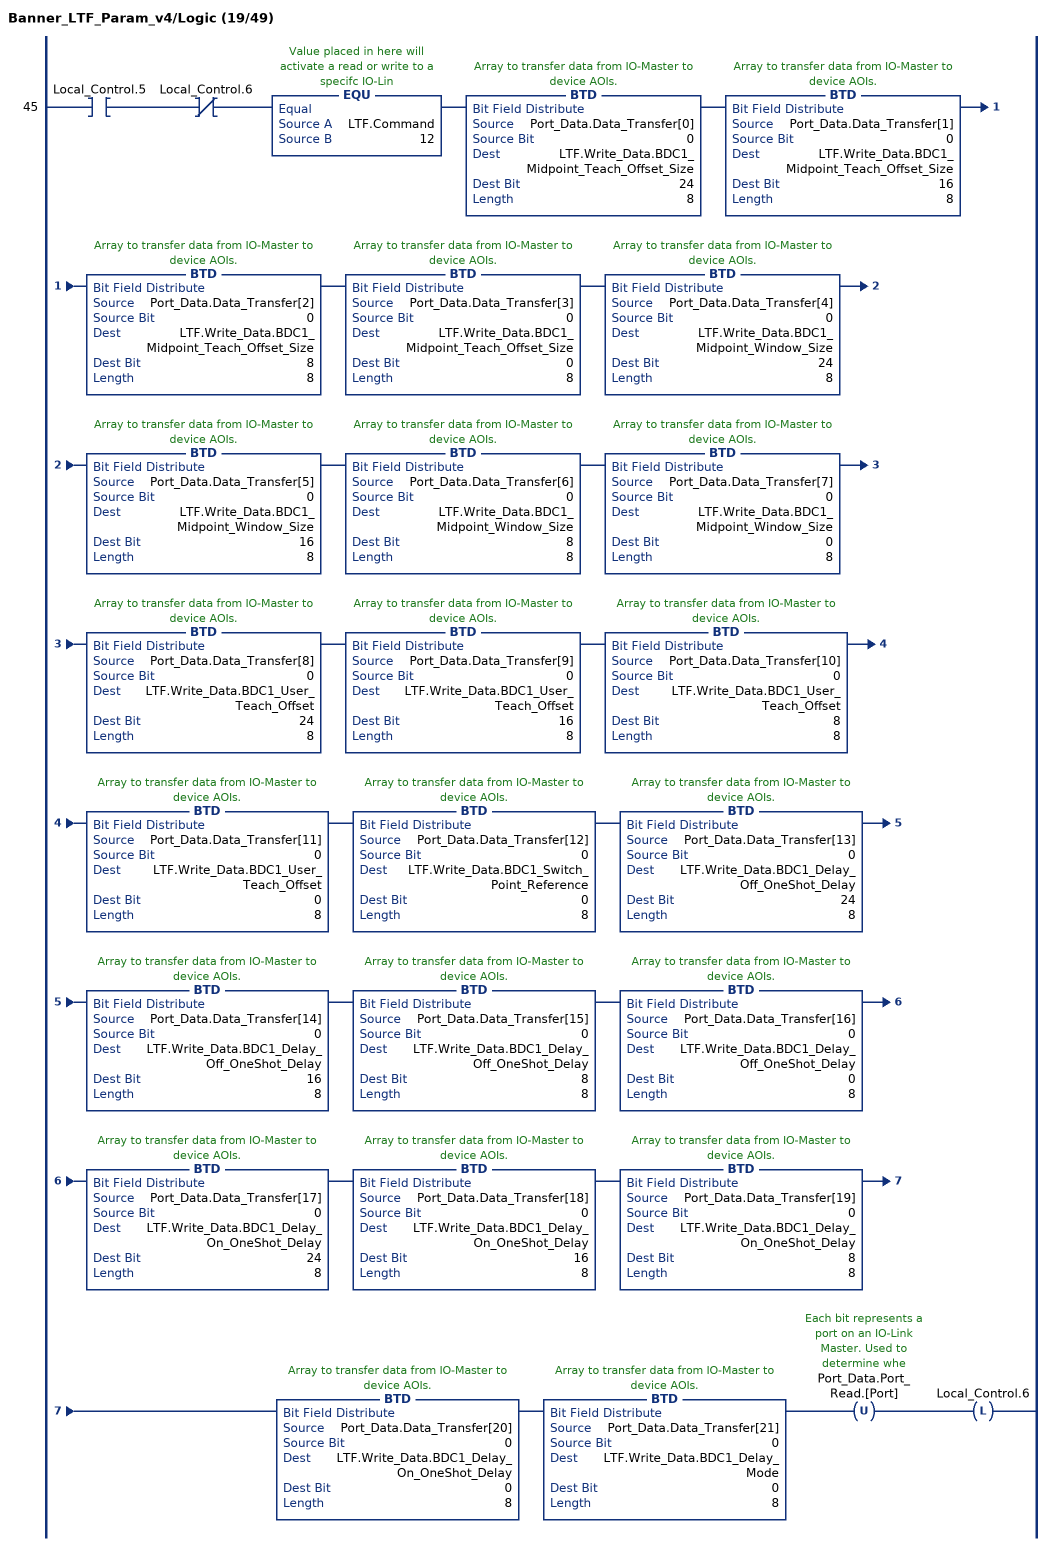
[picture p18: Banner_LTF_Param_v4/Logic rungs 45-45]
   45: XIC(Local_Control.5)XIO(Local_Control.6)EQU(LTF.Command,12)BTD(Port_Data.Data_Transfer[0],0,LTF.Write_Data.BDC1_Midpoint_Teach_Offset_Size,24,8)BTD(Port_Data.Data_Transfer[1],0,LTF.Write_Data.BDC1_Midpoint_Teach_Offset_Size,16,8)BTD(Port_Data.Data_Transfer[2],0,LTF.Write_Data.BDC1_Midpoint_Teach_Offset_Size,8,8)BTD(Port_Data.Data_Transfer[3],0,LTF.Write_Data.BDC1_Midpoint_Teach_Offset_Size,0,8)BTD(Port_Data.Data_Transfer[4],0,LTF.Write_Data.BDC1_Midpoint_Window_Size,24,8)BTD(Port_Data.Data_Transfer[5],0,LTF.Write_Data.BDC1_Midpoint_Window_Size,16,8)BTD(Port_Data.Data_Transfer[6],0,LTF.Write_Data.BDC1_Midpoint_Window_Size,8,8)BTD(Port_Data.Data_Transfer[7],0,LTF.Write_Data.BDC1_Midpoint_Window_Size,0,8)BTD(Port_Data.Data_Transfer[8],0,LTF.Write_Data.BDC1_User_Teach_Offset,24,8)BTD(Port_Data.Data_Transfer[9],0,LTF.Write_Data.BDC1_User_Teach_Offset,16,8)BTD(Port_Data.Data_Transfer[10],0,LTF.Write_Data.BDC1_User_Teach_Offset,8,8)BTD(Port_Data.Data_Transfer[11],0,LTF.Write_Data.BDC1_User_Teach_Offset,0,8)BTD(Port_Data.Data_Transfer[12],0,LTF.Write_Data.BDC1_Switch_Point_Reference,0,8)BTD(Port_Data.Data_Transfer[13],0,LTF.Write_Data.BDC1_Delay_Off_OneShot_Delay,24,8)BTD(Port_Data.Data_Transfer[14],0,LTF.Write_Data.BDC1_Delay_Off_OneShot_Delay,16,8)BTD(Port_Data.Data_Transfer[15],0,LTF.Write_Data.BDC1_Delay_Off_OneShot_Delay,8,8)BTD(Port_Data.Data_Transfer[16],0,LTF.Write_Data.BDC1_Delay_Off_OneShot_Delay,0,8)BTD(Port_Data.Data_Transfer[17],0,LTF.Write_Data.BDC1_Delay_On_OneShot_Delay,24,8)BTD(Port_Data.Data_Transfer[18],0,LTF.Write_Data.BDC1_Delay_On_OneShot_Delay,16,8)BTD(Port_Data.Data_Transfer[19],0,LTF.Write_Data.BDC1_Delay_On_OneShot_Delay,8,8)BTD(Port_Data.Data_Transfer[20],0,LTF.Write_Data.BDC1_Delay_On_OneShot_Delay,0,8)BTD(Port_Data.Data_Transfer[21],0,LTF.Write_Data.BDC1_Delay_Mode,0,8)OTU(Port_Data.Port_Read.[Port])OTL(Local_Control.6);
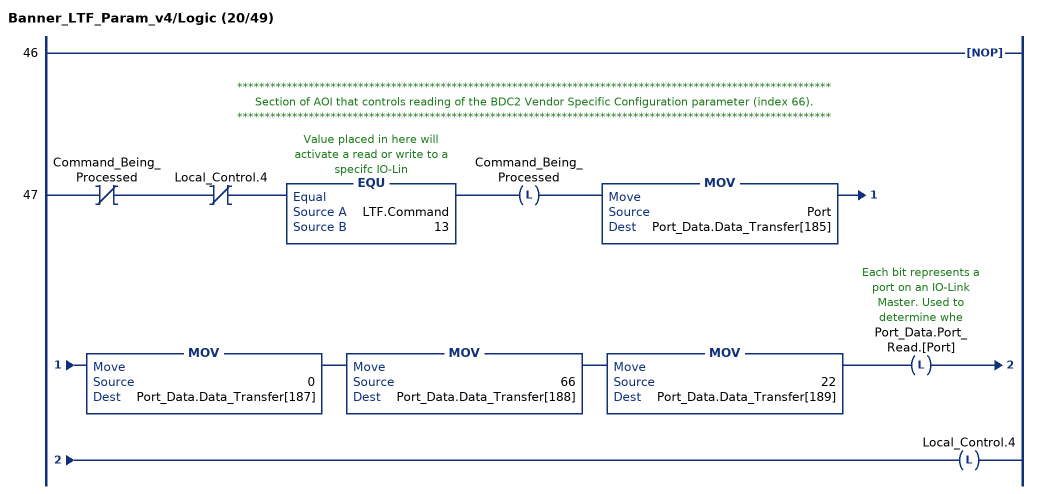
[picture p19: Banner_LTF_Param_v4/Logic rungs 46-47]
   46: NOP();
   // ************************************************************************************************************
   // Section of AOI that controls reading of the BDC2 Vendor Specific Configuration parameter (index 66).
   // ************************************************************************************************************
   47: XIO(Command_Being_Processed)XIO(Local_Control.4)EQU(LTF.Command,13)OTL(Command_Being_Processed)MOV(Port,Port_Data.Data_Transfer[185])MOV(0,Port_Data.Data_Transfer[187])MOV(66,Port_Data.Data_Transfer[188])MOV(22,Port_Data.Data_Transfer[189])OTL(Port_Data.Port_Read.[Port])OTL(Local_Control.4);
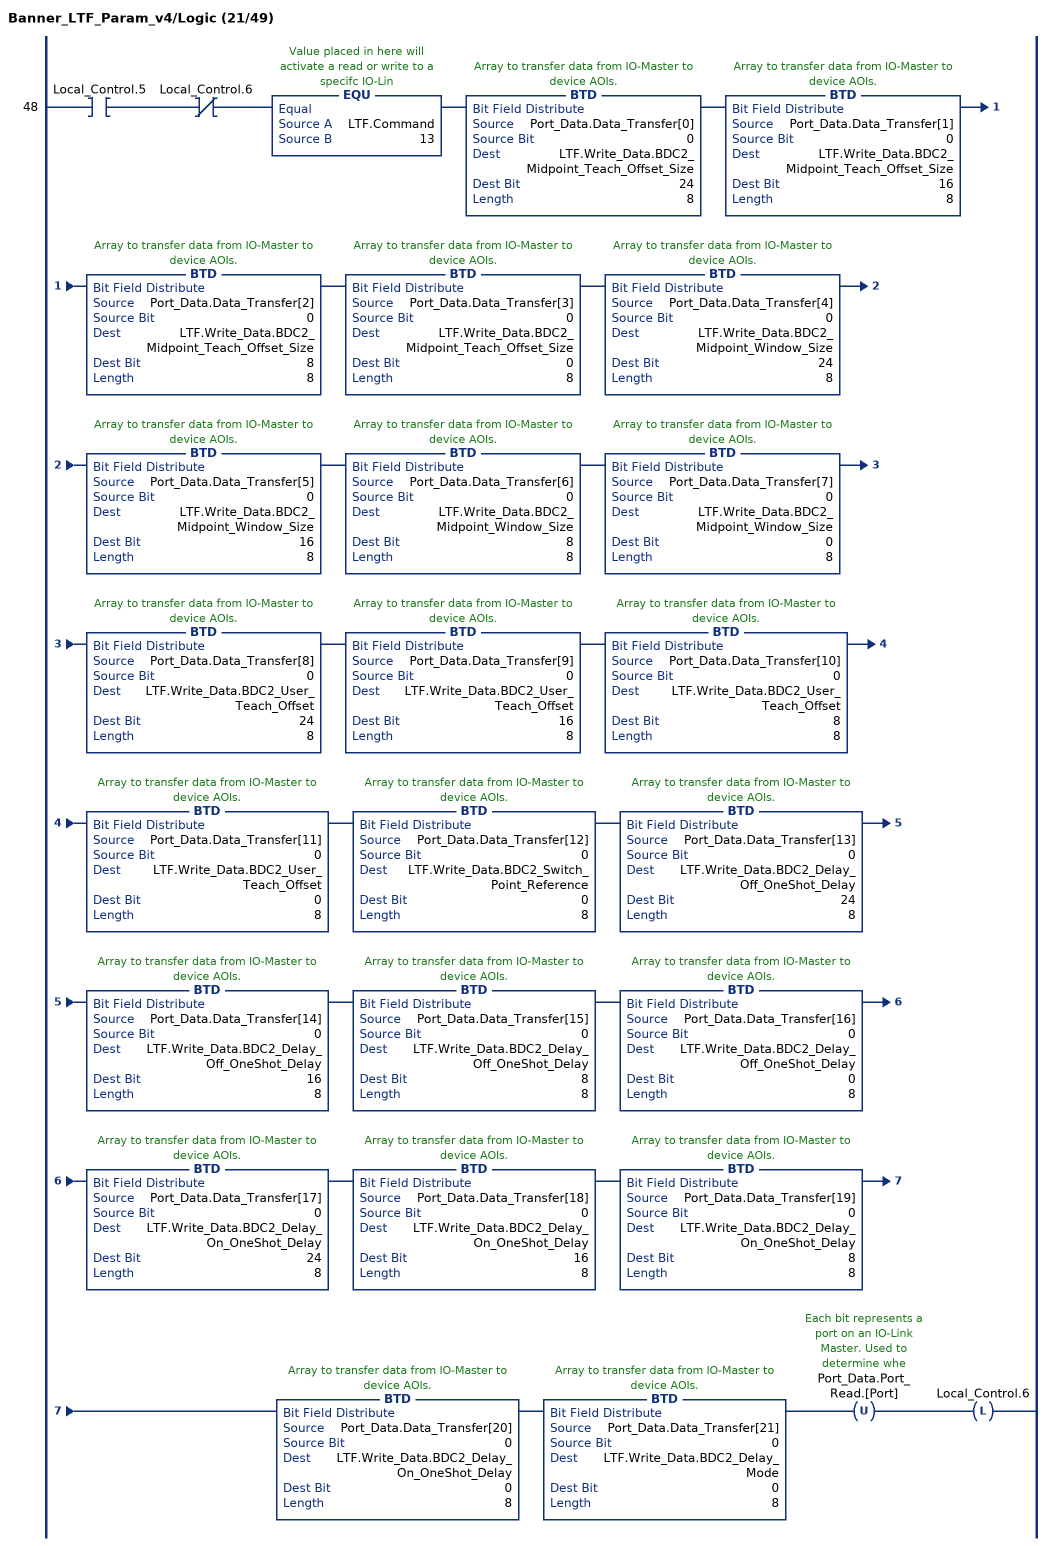
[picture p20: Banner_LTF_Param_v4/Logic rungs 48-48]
   48: XIC(Local_Control.5)XIO(Local_Control.6)EQU(LTF.Command,13)BTD(Port_Data.Data_Transfer[0],0,LTF.Write_Data.BDC2_Midpoint_Teach_Offset_Size,24,8)BTD(Port_Data.Data_Transfer[1],0,LTF.Write_Data.BDC2_Midpoint_Teach_Offset_Size,16,8)BTD(Port_Data.Data_Transfer[2],0,LTF.Write_Data.BDC2_Midpoint_Teach_Offset_Size,8,8)BTD(Port_Data.Data_Transfer[3],0,LTF.Write_Data.BDC2_Midpoint_Teach_Offset_Size,0,8)BTD(Port_Data.Data_Transfer[4],0,LTF.Write_Data.BDC2_Midpoint_Window_Size,24,8)BTD(Port_Data.Data_Transfer[5],0,LTF.Write_Data.BDC2_Midpoint_Window_Size,16,8)BTD(Port_Data.Data_Transfer[6],0,LTF.Write_Data.BDC2_Midpoint_Window_Size,8,8)BTD(Port_Data.Data_Transfer[7],0,LTF.Write_Data.BDC2_Midpoint_Window_Size,0,8)BTD(Port_Data.Data_Transfer[8],0,LTF.Write_Data.BDC2_User_Teach_Offset,24,8)BTD(Port_Data.Data_Transfer[9],0,LTF.Write_Data.BDC2_User_Teach_Offset,16,8)BTD(Port_Data.Data_Transfer[10],0,LTF.Write_Data.BDC2_User_Teach_Offset,8,8)BTD(Port_Data.Data_Transfer[11],0,LTF.Write_Data.BDC2_User_Teach_Offset,0,8)BTD(Port_Data.Data_Transfer[12],0,LTF.Write_Data.BDC2_Switch_Point_Reference,0,8)BTD(Port_Data.Data_Transfer[13],0,LTF.Write_Data.BDC2_Delay_Off_OneShot_Delay,24,8)BTD(Port_Data.Data_Transfer[14],0,LTF.Write_Data.BDC2_Delay_Off_OneShot_Delay,16,8)BTD(Port_Data.Data_Transfer[15],0,LTF.Write_Data.BDC2_Delay_Off_OneShot_Delay,8,8)BTD(Port_Data.Data_Transfer[16],0,LTF.Write_Data.BDC2_Delay_Off_OneShot_Delay,0,8)BTD(Port_Data.Data_Transfer[17],0,LTF.Write_Data.BDC2_Delay_On_OneShot_Delay,24,8)BTD(Port_Data.Data_Transfer[18],0,LTF.Write_Data.BDC2_Delay_On_OneShot_Delay,16,8)BTD(Port_Data.Data_Transfer[19],0,LTF.Write_Data.BDC2_Delay_On_OneShot_Delay,8,8)BTD(Port_Data.Data_Transfer[20],0,LTF.Write_Data.BDC2_Delay_On_OneShot_Delay,0,8)BTD(Port_Data.Data_Transfer[21],0,LTF.Write_Data.BDC2_Delay_Mode,0,8)OTU(Port_Data.Port_Read.[Port])OTL(Local_Control.6);
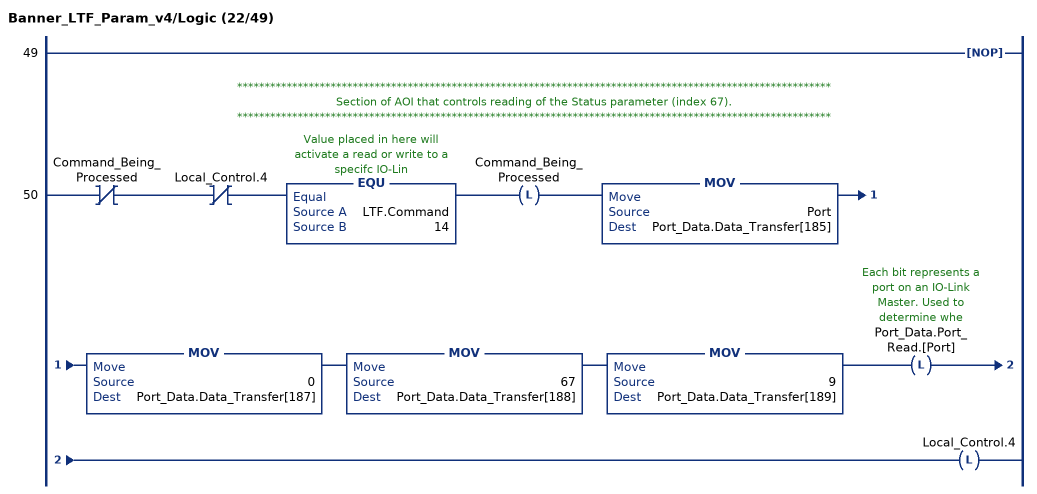
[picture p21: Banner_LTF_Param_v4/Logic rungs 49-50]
   49: NOP();
   // ************************************************************************************************************
   // Section of AOI that controls reading of the Status parameter (index 67).
   // ************************************************************************************************************
   50: XIO(Command_Being_Processed)XIO(Local_Control.4)EQU(LTF.Command,14)OTL(Command_Being_Processed)MOV(Port,Port_Data.Data_Transfer[185])MOV(0,Port_Data.Data_Transfer[187])MOV(67,Port_Data.Data_Transfer[188])MOV(9,Port_Data.Data_Transfer[189])OTL(Port_Data.Port_Read.[Port])OTL(Local_Control.4);
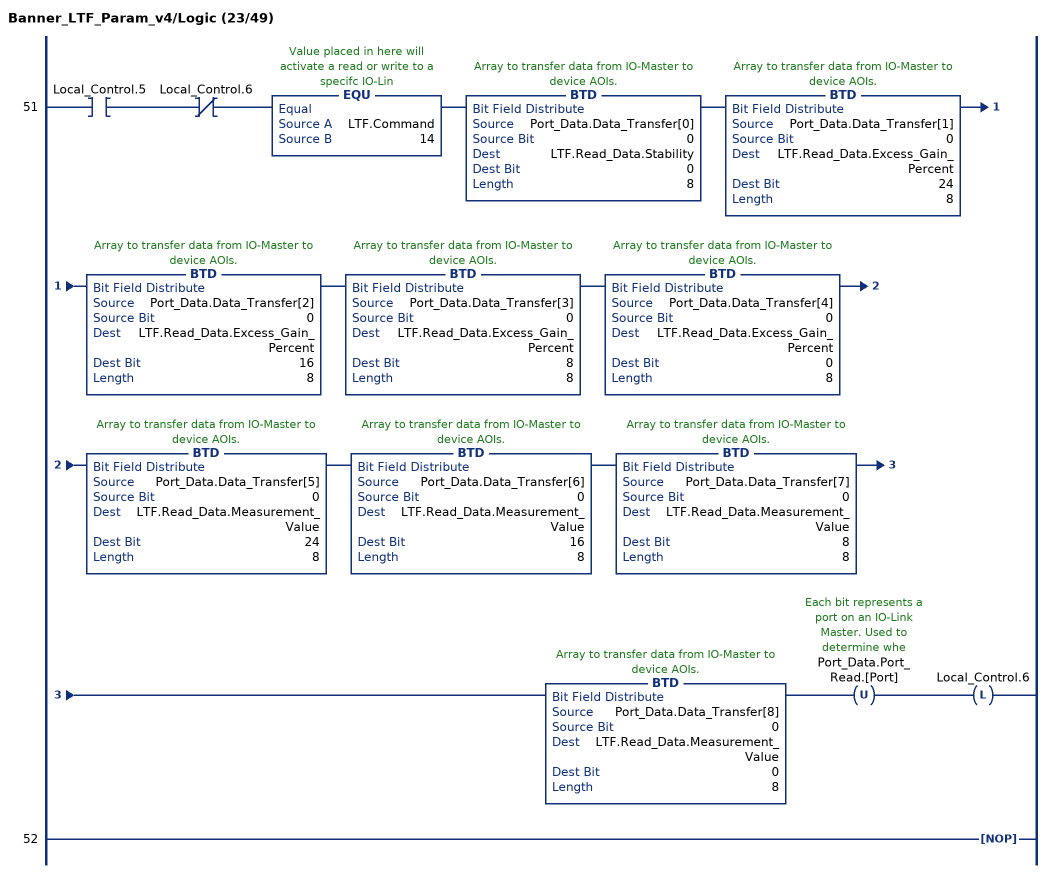
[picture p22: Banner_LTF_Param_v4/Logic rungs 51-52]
   51: XIC(Local_Control.5)XIO(Local_Control.6)EQU(LTF.Command,14)BTD(Port_Data.Data_Transfer[0],0,LTF.Read_Data.Stability,0,8)BTD(Port_Data.Data_Transfer[1],0,LTF.Read_Data.Excess_Gain_Percent,24,8)BTD(Port_Data.Data_Transfer[2],0,LTF.Read_Data.Excess_Gain_Percent,16,8)BTD(Port_Data.Data_Transfer[3],0,LTF.Read_Data.Excess_Gain_Percent,8,8)BTD(Port_Data.Data_Transfer[4],0,LTF.Read_Data.Excess_Gain_Percent,0,8)BTD(Port_Data.Data_Transfer[5],0,LTF.Read_Data.Measurement_Value,24,8)BTD(Port_Data.Data_Transfer[6],0,LTF.Read_Data.Measurement_Value,16,8)BTD(Port_Data.Data_Transfer[7],0,LTF.Read_Data.Measurement_Value,8,8)BTD(Port_Data.Data_Transfer[8],0,LTF.Read_Data.Measurement_Value,0,8)OTU(Port_Data.Port_Read.[Port])OTL(Local_Control.6);
   52: NOP();
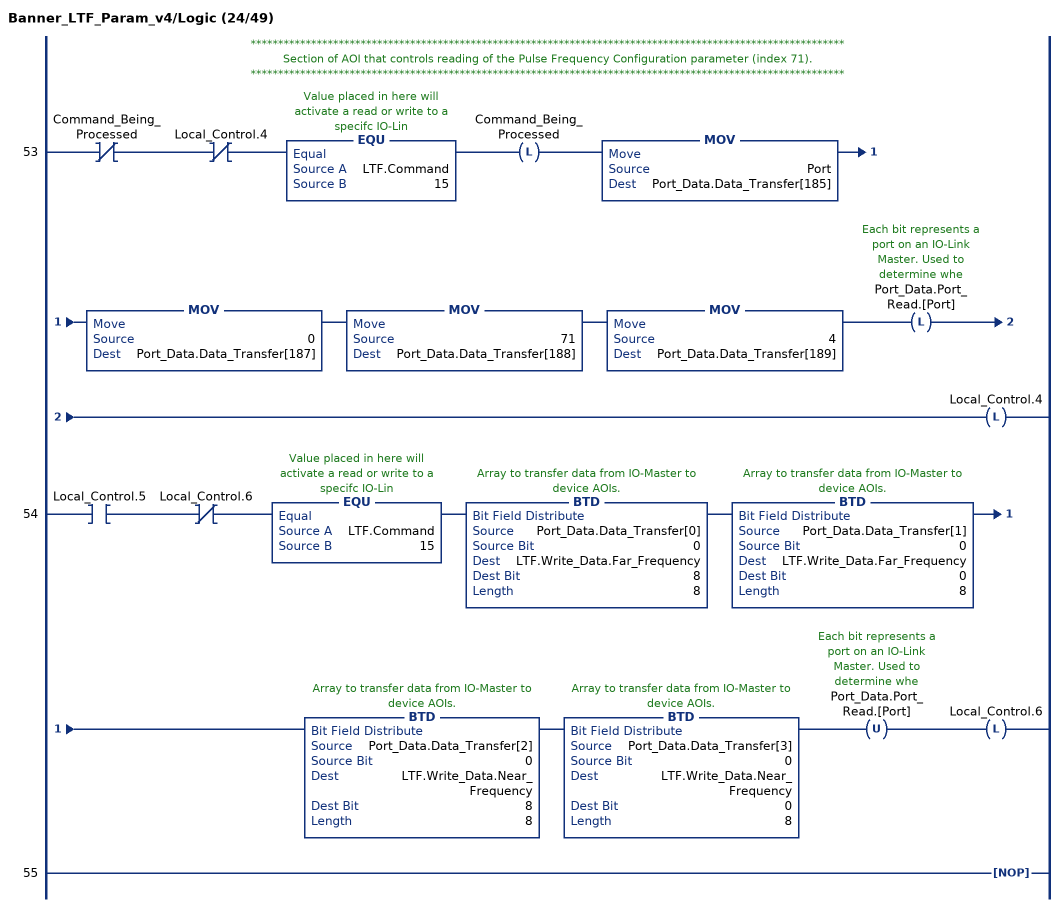
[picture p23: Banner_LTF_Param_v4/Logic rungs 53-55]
   // ************************************************************************************************************
   // Section of AOI that controls reading of the Pulse Frequency Configuration parameter (index 71).
   // ************************************************************************************************************
   53: XIO(Command_Being_Processed)XIO(Local_Control.4)EQU(LTF.Command,15)OTL(Command_Being_Processed)MOV(Port,Port_Data.Data_Transfer[185])MOV(0,Port_Data.Data_Transfer[187])MOV(71,Port_Data.Data_Transfer[188])MOV(4,Port_Data.Data_Transfer[189])OTL(Port_Data.Port_Read.[Port])OTL(Local_Control.4);
   54: XIC(Local_Control.5)XIO(Local_Control.6)EQU(LTF.Command,15)BTD(Port_Data.Data_Transfer[0],0,LTF.Write_Data.Far_Frequency,8,8)BTD(Port_Data.Data_Transfer[1],0,LTF.Write_Data.Far_Frequency,0,8)BTD(Port_Data.Data_Transfer[2],0,LTF.Write_Data.Near_Frequency,8,8)BTD(Port_Data.Data_Transfer[3],0,LTF.Write_Data.Near_Frequency,0,8)OTU(Port_Data.Port_Read.[Port])OTL(Local_Control.6);
   55: NOP();
